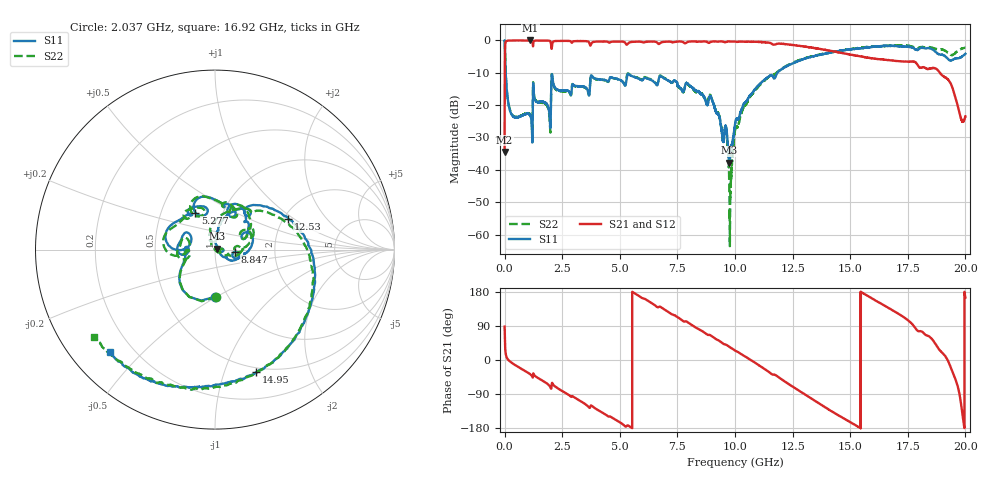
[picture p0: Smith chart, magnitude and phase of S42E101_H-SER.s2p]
!{S42E101}
!Johanson Technology Inc.
!www.johansontechnology.com
!Test Board Conditions:
!Substrate Type  RO4350B
!Substrate Thickness  50 mil
!Substrate Dk  3.66
!TL Type: GCPW
!TL Trace Width  60 mil
!TL Gap  10 mil
!Electrode orientation  Horizontal
!DUT TOPOLOGY	SERIES
!Mounting Pad LxW  14x55 mil
! Created Wed Nov 25 21:53:21 2020
# khz S ma R 50
! 2 Port Network Data from SP1.SP block
! freq  magS11  angS11  magS21  angS21  magS12  angS12  magS22  angS22
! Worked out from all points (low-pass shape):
!   20001 points, 300 kHz to 20 GHz, reference 50 ohm
!   highest |S21| = -0.03 dB at 1.123 GHz (marker M1); lowest = -34.5 dB at 300 kHz (marker M2)
!   |S21| within 3 dB of the highest: 15.88 MHz to 13.97 GHz (13.96 GHz wide, 200 % of centre); 13.97628 GHz to 13.9918 GHz (15.52 MHz wide, 0.111 % of centre)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
!   lowest |S11| = -37.8 dB at 9.759 GHz (marker M3), VSWR 1.03, Z = 51.2 + j0.521 ohm
!   |S11| at or under -10 dB: 47.83 MHz to 11.84 GHz (11.79 GHz wide, 198 % of centre)
!   |S22| runs from -63.6 to 0.0 dB; largest |S21 - S12| = 0.017
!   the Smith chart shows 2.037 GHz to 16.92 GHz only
!   S11 on the Smith chart (normalised r, x): 2.037 GHz: 0.87, -0.49; 5.277 GHz: 0.74, +0.32; 8.847 GHz: 1.25, -0.03; 12.53 GHz: 2.12, +0.90; 14.95 GHz: 0.45, -1.29; 16.92 GHz: 0.12, -0.40
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300  0.9951 -1.1  0.0188 88.0  0.01899 88.6  0.9936 -1.2
115300  0.143 -86.7  0.9884 3.9  0.9877 3.9  0.1439 -86.7
349300  0.06813 -100.6  0.9957 -9.2  0.9961 -9.1  0.06928 -100.5
1123300  0.06806 -129.8  0.997 -37.9  0.9959 -37.9  0.06976 -127.1
1321300  0.1199 -133.5  0.9901 -42.2  0.9889 -42.2  0.1226 -130.3
1909300  0.08816 -151.1  0.9881 -65.4  0.989 -65.5  0.08376 -153.3
2037300  0.2622 -89.7  0.7438 -70.0  0.7437 -70.1  0.2643 -88.4
3334300  0.1952 155.7  0.975 -110.0  0.9751 -110.0  0.1924 164.3
5277300  0.2322 117.9  0.8679 -175.4  0.8682 -175.4  0.2415 122.1
6667300  0.2285 72.5  0.8875 139.2  0.8849 139.1  0.2304 69.3
8847300  0.1136 -6.0  0.9175 66.0  0.9178 66.0  0.1274 9.1
9616300  0.04494 -12.9  0.9428 40.3  0.9444 40.2  0.04231 -16.0
9759300  0.0129 23.2  0.9637 34.4  0.9639 34.3  0.004005 -60.4
1.00003e7  0.05012 86.0  0.9578 24.9  0.9585 24.9  0.04095 120.6
1.11213e7  0.2194 67.4  0.9433 -17.2  0.939 -17.3  0.2115 74.8
1.25303e7  0.4435 22.7  0.8474 -71.4  0.8471 -71.2  0.4556 14.3
1.33343e7  0.5593 -8.7  0.7725 -102.4  0.7763 -102.3  0.5671 -15.6
1.49523e7  0.7202 -71.5  0.6104 -162.1  0.6076 -162.8  0.7297 -73.2
1.66673e7  0.8193 -126.8  0.4977 137.4  0.485 137.8  0.8265 -136.0
1.69193e7  0.8196 -136.1  0.4846 128.3  0.4722 128.9  0.8297 -144.2
1.87963e7  0.6236 150.5  0.3488 33.5  0.3487 33.1  0.729 159.9
2e7  0.62 149.4  0.0666 164.9  0.06678 165.0  0.7686 123.7
